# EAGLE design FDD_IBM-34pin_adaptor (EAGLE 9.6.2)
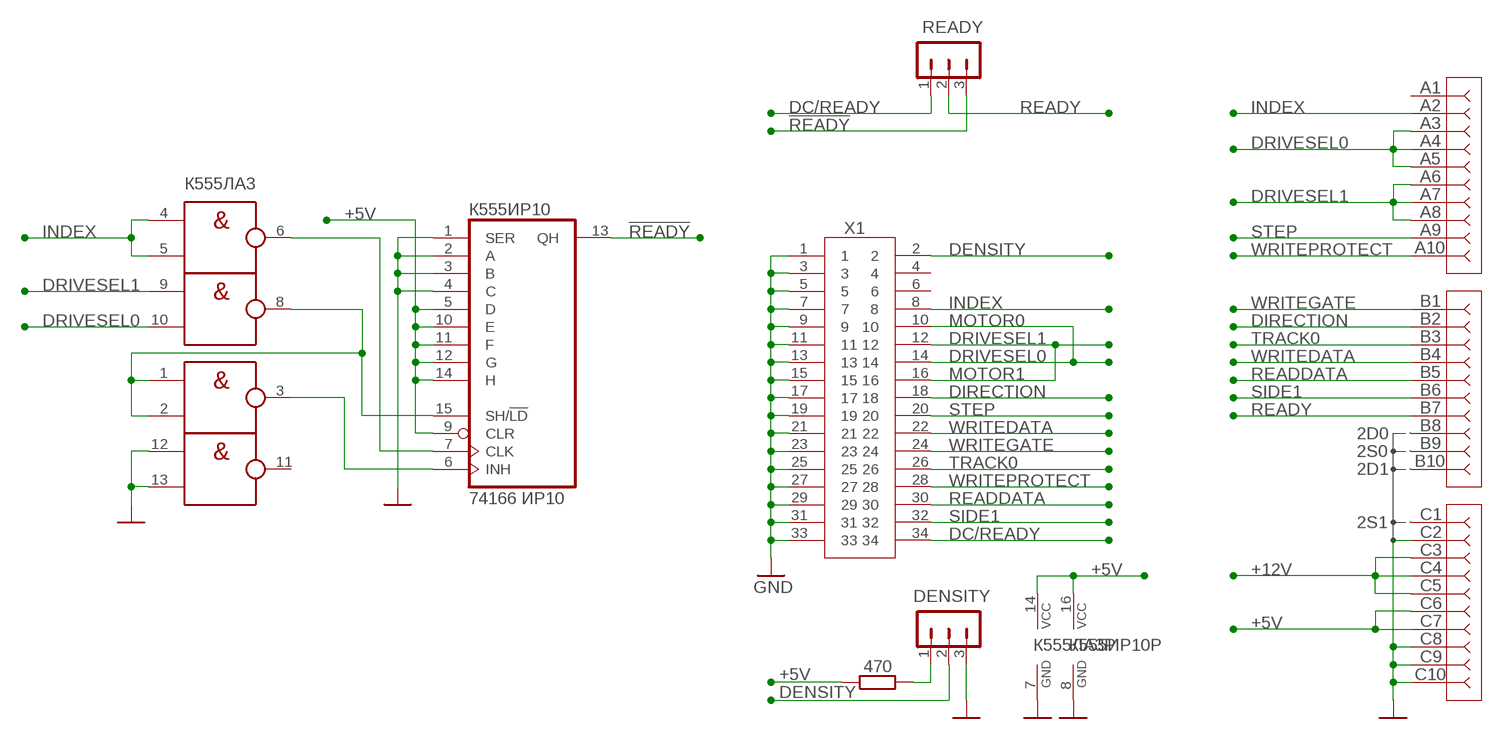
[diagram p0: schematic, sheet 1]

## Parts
DENSITY  JP3S  [JP3S]
R1  470  R-EU_0207/7  [0207/7]
READY  JP3S  [JP3S]
U$2  FDD-30PIN  [FDD-30PIN]
X1  057-034-B  [057-034-1]
К555ИР10  74166 ИР10  74HC166N  [DIL16]
К555ЛА3  К555ЛА3  74LS00N  [DIL14]

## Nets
2D0: U$2.B8
2D1: U$2.B10
2S0: U$2.B9
2S1: U$2.C1
!READY: READY.3 К555ИР10.13(QH)
+5V: R1.1 U$2.C6 U$2.C7 К555ИР10.5(D) К555ИР10.9(CLR) К555ИР10.10(E) К555ИР10.11(F) К555ИР10.12(G) К555ИР10.14(H) К555ИР10.16(VCC) К555ЛА3.14(P:VCC)
+12V: U$2.C3 U$2.C4 U$2.C5
DC/READY: READY.1 X1.34
DENSITY: DENSITY.2 X1.2
DIRECTION: U$2.B2 X1.18
DRIVESEL0: U$2.A3 U$2.A4 U$2.A5 X1.10 X1.14 К555ЛА3.10(C:I1)
DRIVESEL1: U$2.A6 U$2.A7 U$2.A8 X1.12 X1.16 К555ЛА3.9(C:I0)
GND: DENSITY.3 U$2.C2 U$2.C8 U$2.C9 U$2.C10 X1.1 X1.3 X1.5 X1.7 X1.9 X1.11 X1.13 X1.15 X1.17 X1.19 X1.21 X1.23 X1.25 X1.27 X1.29 X1.31 X1.33 К555ИР10.1(SER) К555ИР10.2(A) К555ИР10.3(B) К555ИР10.4(C) К555ИР10.8(GND) К555ЛА3.7(P:GND) К555ЛА3.12(D:I0) К555ЛА3.13(D:I1)
INDEX: U$2.A2 X1.8 К555ЛА3.4(B:I0) К555ЛА3.5(B:I1)
N$1: DENSITY.1 R1.2
N$3: К555ИР10.15(SH/!LD) К555ЛА3.1(A:I0) К555ЛА3.2(A:I1) К555ЛА3.8(C:O)
N$4: К555ИР10.6(INH) К555ЛА3.3(A:O)
N$5: К555ИР10.7(CLK) К555ЛА3.6(B:O)
READDATA: U$2.B5 X1.30
READY: READY.2 U$2.B7
SIDE1: U$2.B6 X1.32
STEP: U$2.A9 X1.20
TRACK0: U$2.B3 X1.26
WRITEDATA: U$2.B4 X1.22
WRITEGATE: U$2.B1 X1.24
WRITEPROTECT: U$2.A10 X1.28
Unconnected: U$2.A1 X1.4 X1.6 К555ЛА3.11(D:O)

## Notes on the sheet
- MOTOR0
- MOTOR1

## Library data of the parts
DENSITY READY = jumpers_lib:JP3S
R1 = rcl:R-EU_: RESISTOR, European symbol; SPICEPREFIX: R
U$2 = AGAT_Slot_Connector:FDD-30PIN
X1 = con-panduit:057-034-: CONNECTOR 34-pin series 057 contact pc board low profile headers
К555ИР10 = 74xx-eu:74*166: 8-bit parallel load SHIFT REGISTER
К555ЛА3 = 74xx-eu:74*00: Quad 2-input NAND gate

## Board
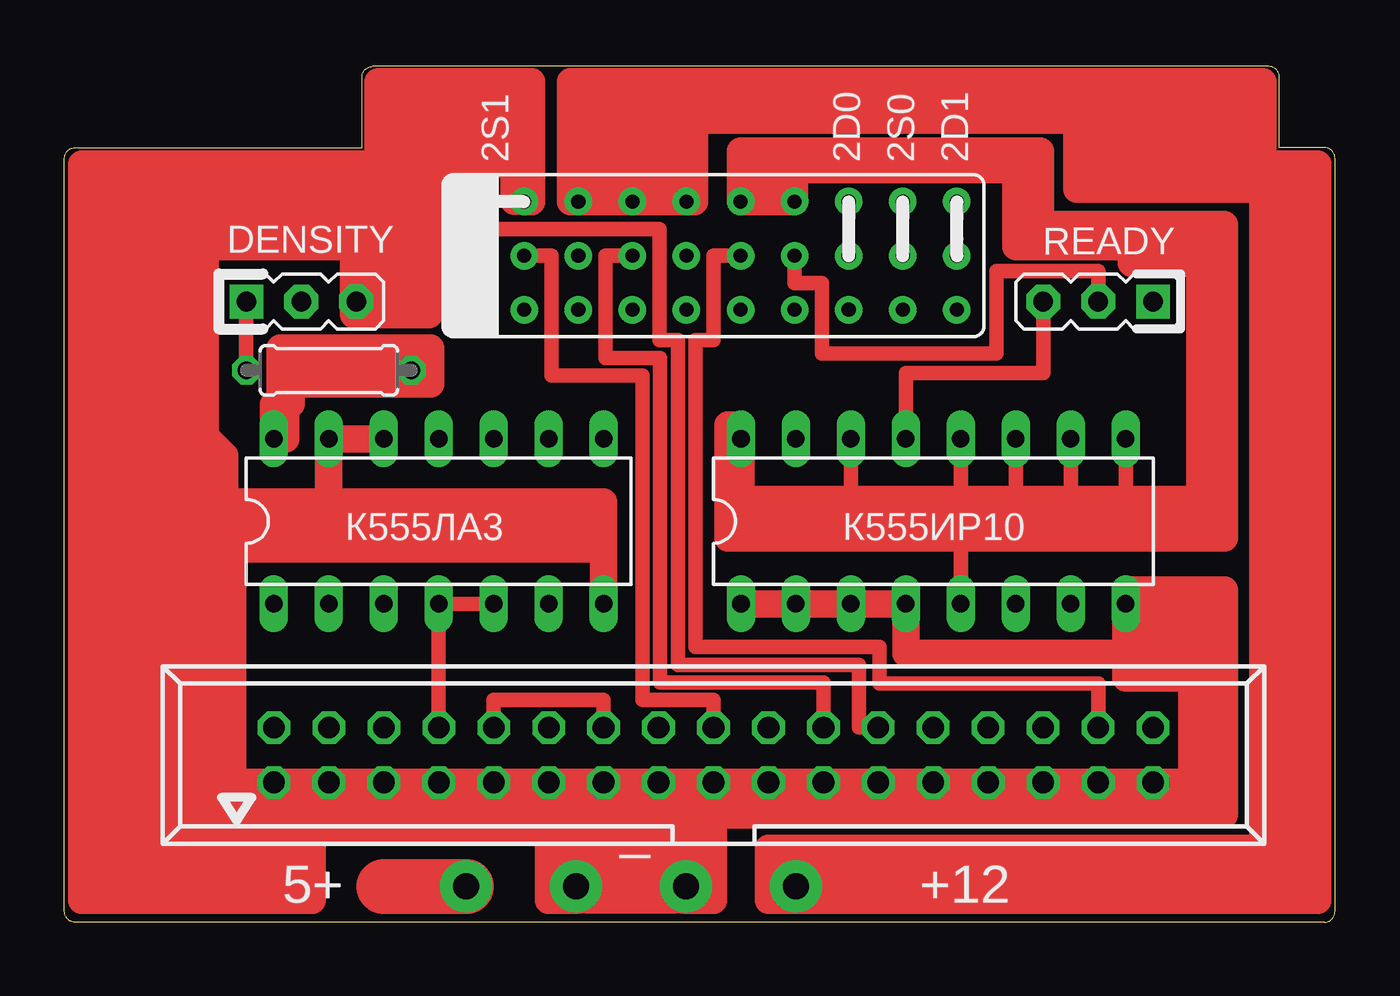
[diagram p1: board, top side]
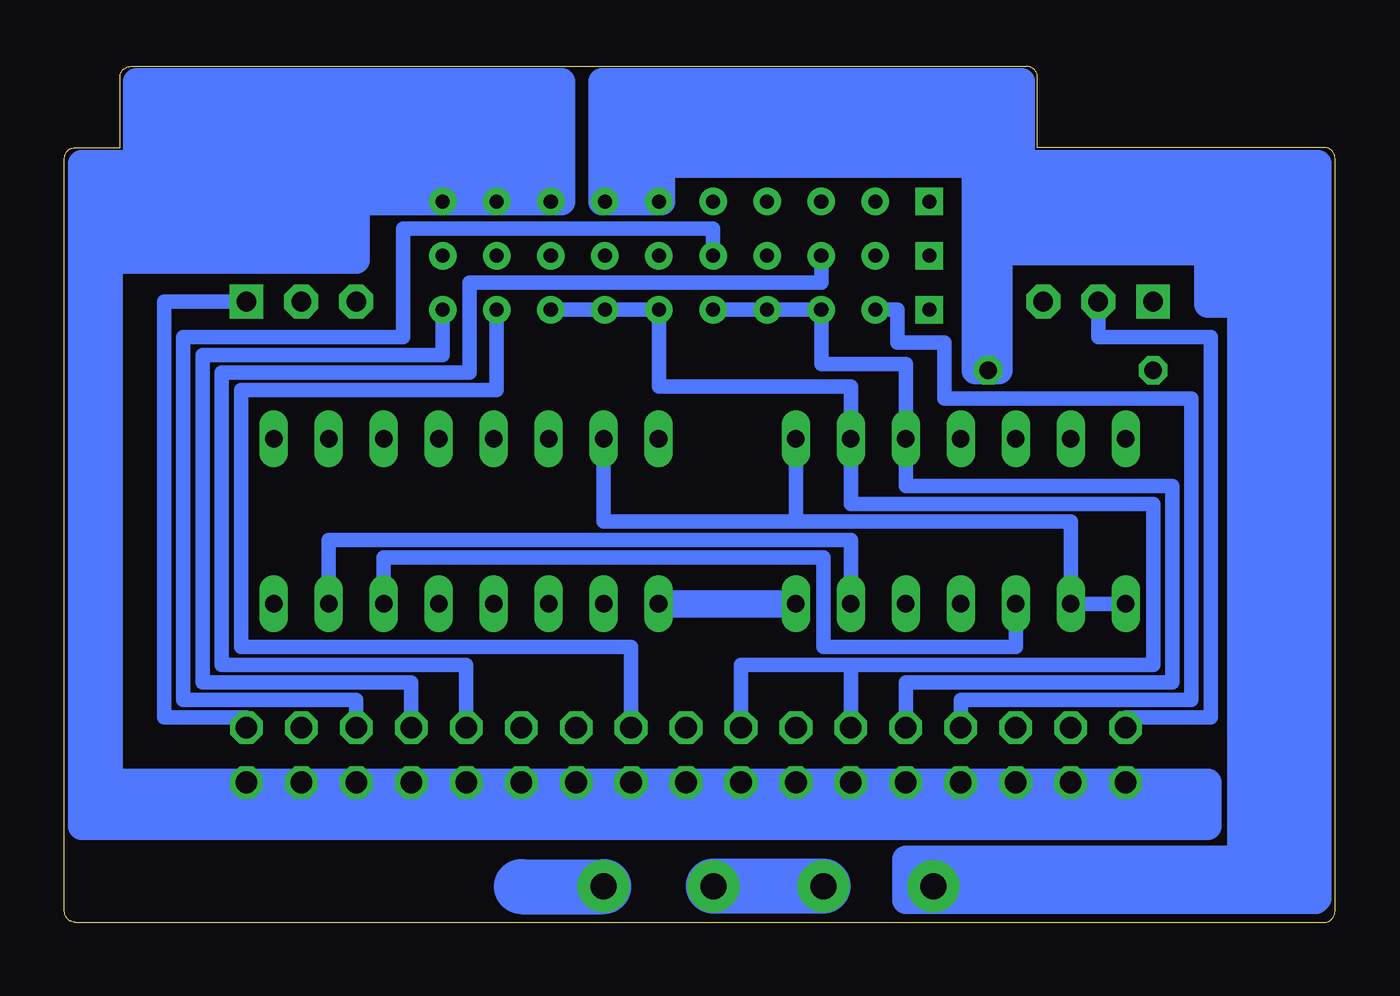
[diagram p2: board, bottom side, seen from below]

Size 58.73 x 39.56 mm. Coordinates in mm from the lower left corner, seen from the top.
Outline: 58.23,0 0.5,0 arc-90 0,0.5 0,35.31 arc-90 0.5,35.81 13.75,35.81 13.75,39.06 arc-90 14.25,39.56 55.66,39.56 arc-90 56.16,39.06 56.16,35.81 58.23,35.81 arc-90 58.73,35.31 58.73,0.5 arc-90 58.23,0
Copper layers (1*16): Top 0.035mm / dielectric 1.5mm / Bottom 0.035mm
Design rules "default *": minimum track width 6mil, minimum drill 0.35mm, track to track 6mil, track to pad 6mil, pad to pad 6mil, via to via 6mil, smd to smd 6mil, copper to edge 0mil, drill to drill 6mil, minimum pad ring 10mil, minimum via ring 8mil, stop-mask expansion 0mil, vias tented up to drill 0mil, thermal gap 10mil

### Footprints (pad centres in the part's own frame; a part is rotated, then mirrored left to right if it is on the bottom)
JP3S = drill 0.914 pad 1.57 square: 1 -2.54,0 | drill 0.914 pad 1.57 octagon: 2 0,0; 3 2.54,0
0207/7 = drill 0.813 octagon: 1 -3.81,0; 2 3.81,0
FDD-30PIN = drill 0.65 pad 1.27 square: A1 -11.25,-2.5; B1 -11.25,0; C1 -11.25,2.5 | drill 0.65 pad 1.27: A2 -8.75,-2.5; A3 -6.25,-2.5; A4 -3.75,-2.5; A5 -1.25,-2.5; A6 1.25,-2.5; A7 3.75,-2.5; A8 6.25,-2.5; A9 8.75,-2.5; A10 11.25,-2.5; B2 -8.75,0; B3 -6.25,0; B4 -3.75,0; B5 -1.25,0; B6 1.25,0; B7 3.75,0; B8 6.25,0; B9 8.75,0; B10 11.25,0; C2 -8.75,2.5; C3 -6.25,2.5; C4 -3.75,2.5; C5 -1.25,2.5; C6 1.25,2.5; C7 3.75,2.5; C8 6.25,2.5; C9 8.75,2.5; C10 11.25,2.5
057-034-1 = drill 1 octagon: 1 -20.32,-1.27; 2 -20.32,1.27; 3 -17.78,-1.27; 4 -17.78,1.27; 5 -15.24,-1.27; 6 -15.24,1.27; 7 -12.7,-1.27; 8 -12.7,1.27; 9 -10.16,-1.27; 10 -10.16,1.27; 11 -7.62,-1.27; 12 -7.62,1.27; 13 -5.08,-1.27; 14 -5.08,1.27; 15 -2.54,-1.27; 16 -2.54,1.27; 17 0,-1.27; 18 0,1.27; 19 2.54,-1.27; 20 2.54,1.27; 21 5.08,-1.27; 22 5.08,1.27; 23 7.62,-1.27; 24 7.62,1.27; 25 10.16,-1.27; 26 10.16,1.27; 27 12.7,-1.27; 28 12.7,1.27; 29 15.24,-1.27; 30 15.24,1.27; 31 17.78,-1.27; 32 17.78,1.27; 33 20.32,-1.27; 34 20.32,1.27
DIL16 = drill 0.813 long: 1 -8.89,-3.81; 2 -6.35,-3.81; 3 -3.81,-3.81; 4 -1.27,-3.81; 5 1.27,-3.81; 6 3.81,-3.81; 7 6.35,-3.81; 8 8.89,-3.81; 9 8.89,3.81; 10 6.35,3.81; 11 3.81,3.81; 12 1.27,3.81; 13 -1.27,3.81; 14 -3.81,3.81; 15 -6.35,3.81; 16 -8.89,3.81
DIL14 = drill 0.813 long: 1 -7.62,-3.81; 2 -5.08,-3.81; 3 -2.54,-3.81; 4 0,-3.81; 5 2.54,-3.81; 6 5.08,-3.81; 7 7.62,-3.81; 8 7.62,3.81; 9 5.08,3.81; 10 2.54,3.81; 11 0,3.81; 12 -2.54,3.81; 13 -5.08,3.81; 14 -7.62,3.81

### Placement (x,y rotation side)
DENSITY  10.95,28.7 0 top
R1  12.22,25.52 180 top
READY  47.78,28.7 180 top
U$2  30,30.82 0 top
X1  30,7.73 0 top
К555ИР10  40.16,18.54 0 top
К555ЛА3  17.3,18.54 0 top

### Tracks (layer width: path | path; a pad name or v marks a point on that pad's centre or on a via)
2D0
  Top 0.61: 36.26,31.6 U$2.B8
2D1
  Top 0.61: 41.26,31.6 U$2.B10
2S0
  Top 0.61: 38.76,31.6 U$2.B9
2S1
  Top 0.61: 19.54,33.31 U$2.C1
!READY
  Top 0.66: К555ИР10.13 38.89,25.39 45.24,25.39 READY.3
+5V  (via drill 1.2 pad 2.4)
  Top 0.66: К555ИР10.14 36.35,19.55 | К555ИР10.12 41.43,19.55 | К555ИР10.11 43.97,19.55 | К555ИР10.10 46.51,19.55 | К555ИР10.9 49.05,19.55 | К555ИР10.5 41.43,17.77
  Top 1.27: 52.48,30.47 52.48,31.24 49.3,31.24 | 52.48,30.47 52.48,19.55 49.05,19.55 46.51,19.55 43.97,19.55 41.43,19.55 36.35,19.55 31.27,19.55 | 31.27,19.55 31.27,18.66 | 53.62,18.66 31.27,18.66 | 31.25,35.66 U$2.C6 32.16,33.31 | 31.25,35.66 33.05,35.66 | 33.05,35.66 45.11,35.66 45.11,32.25 53.62,32.25 53.62,18.66 | 32.16,33.31 33.05,33.31 | 33.05,33.31 U$2.C7 33.75,34.79 43.97,34.79 43.97,31.24 49.3,31.24 | 33.05,35.66 33.05,33.31 | 31.25,35.66 32.16,34.75 32.16,33.31 | 31.27,18.66 31.27,17.77 | 53.62,18.66 53.62,17.77 41.43,17.77 31.27,17.77 | 49.3,31.24 49.3,30.47 52.48,30.47 | 10.21,23.97 10.47,23.97 10.47,24.89 | 10.21,23.97 9.96,23.97 | 10.47,24.89 10.47,25.52 R1.1 | R1.1 16.03,24.89 | 16.03,24.89 10.47,24.89 | R1.1 16.92,25.52 | 16.92,25.52 16.92,24.89 16.03,24.89 | 16.92,25.52 16.92,26.54 9.96,26.54 9.96,23.97 | 9.96,23.97 9.68,23.97 К555ЛА3.14 10.21,22.35 10.21,23.97 | 31.27,19.55 К555ИР10.16 31.27,22.98 30.66,22.98 30.66,17.77 31.27,17.77
  Bottom 1.27: 31.93,33.31 U$2.C6 31.12,33.31 31.12,35.05 16.62,35.05 16.62,31 | 31.93,33.31 32.83,33.31 | 32.83,33.31 U$2.C7 33.88,33.31 33.88,38.87 14.5,38.87 14.5,37.86 | 3.99,32 3.99,34.24 | 2.72,34.24 2.72,35.06 | 3.99,34.24 2.72,34.24 | 2.72,34.24 1.83,34.24 1.83,32.97 1.96,32.97 | 10.09,32.97 3.2,32.97 | 10.09,32.97 10.09,33.14 | 10.09,33.14 10.09,34.12 | 10.09,34.12 10.09,34.24 | 10.09,34.24 10.09,35.06 | 3.99,34.24 6.53,34.24 | 6.53,34.24 10.09,34.24 | 2.72,35.06 6.53,35.06 | 6.53,35.06 10.09,35.06 | 31.93,35.93 31.93,33.31 | 32.83,33.31 32.83,37.86 14.5,37.86 | 6.53,35.06 6.53,34.24 | 10.09,32.97 10.09,32 | 14.5,36.94 14.5,35.93 | 14.5,36.94 14.5,37.86 | 14.5,36.94 31.93,36.94 31.93,35.93 | 31.93,35.93 15.64,35.93 | 15.64,35.93 14.5,35.93 | 16.62,31 15.64,31 15.64,35.93 | 10.09,32 4.6,32 | 4.6,32 3.99,32 | 3.99,32 3.48,32 3.48,31 3.96,31 | 14.62,34.12 14.62,35.06 14.5,35.06 | 14.62,34.12 14.62,33.14 | 14.62,33.14 14.62,32 | 14.62,32 14.62,31 | 10.09,34.12 14.62,34.12 | 14.62,32 10.09,32 | 14.62,33.14 10.09,33.14 | 10.09,35.06 14.5,35.06 | 14.5,35.06 14.5,35.93 | 5.87,31 14.62,31 | 5.87,31 3.96,31 | 19.84,1.66 v18.57,1.66 | 2.72,35.06 0.79,35.06 0.79,1.11 0.88,1.02 19.84,1.02 19.84,1.66 | 1.96,32.97 1.96,1.9 19.84,1.9 | 19.84,1.9 19.84,1.66 | 19.84,1.9 19.84,2.64 | 1.96,32.97 3.2,32.97 | 19.84,2.64 19.84,2.91 3.08,2.91 3.08,28.7 3.2,28.7 | 19.84,2.64 4.35,2.64 4.35,28.57 4.6,28.57 | 3.96,26.54 3.96,27.43 3.2,27.43 3.2,28.7 | 3.2,28.7 3.2,32.97 | 5.87,31 5.87,28.57 4.6,28.57 | 3.96,31 3.96,28.7 | 3.96,28.7 3.96,27.55 | 3.96,28.7 3.2,28.7 | 16.62,31 16.62,27.43 | 14.62,31 15.54,31 15.54,27.43 | 15.54,27.43 16.62,27.43 | 16.62,27.43 16.62,25.52 R1.1 15.54,25.52 15.54,27.43
  Bottom 1.27: 4.6,32 4.6,28.57
+12V  (via drill 1.2 pad 2.4)
  Top 1.27: 27.87,33.31 U$2.C5 29.11,33.31 29.11,37.84 | 27.87,33.31 26.85,33.31 | 26.85,33.31 U$2.C4 | U$2.C4 25.33,33.31 | 25.33,33.31 24.56,33.31 | 24.56,33.31 U$2.C3 | 24.56,33.31 24.56,36.7 | 24.56,36.7 25.33,36.7 | 25.33,33.31 25.33,36.7 | 26.85,33.31 26.85,36.7 | 26.85,36.7 26.25,36.7 | 26.25,36.7 25.33,36.7 | 23.75,36.7 24.56,36.7 | U$2.C3 23.75,36.7 | 26.85,36.7 27.87,36.7 | 27.87,36.7 27.87,37.08 46.79,37.08 | 27.87,36.7 27.87,33.31 | 23.75,37.84 23.75,36.7 | 23.75,37.84 23.75,38.85 | 46.79,37.08 55.4,37.08 | U$2.C4 26.25,36.7 | U$2.C3 23.4,33.32 23.4,38.85 23.75,38.85 | 23.75,37.84 29.11,37.84 | 55.4,37.84 55.4,37.08 | 23.75,38.85 55.4,38.85 55.4,37.84 | 29.11,37.84 55.4,37.84 | 55.4,37.08 55.4,36.06 | 55.4,36.06 55.4,35.05 | 55.4,35.05 56.67,35.05 | 56.67,35.05 57.94,35.05 57.94,3.42 | 57.94,2.91 57.94,1.64 | 57.94,1.64 57.94,1.02 32.54,1.02 32.54,1.64 | 32.54,1.64 32.54,3.42 33.56,3.42 33.56,1.92 v33.81,1.66 | 33.81,2.91 55.4,2.91 | 55.4,2.91 56.67,2.91 | 56.67,2.91 57.94,2.91 | 57.94,3.42 57.94,2.91 | v33.81,1.66 33.79,1.64 32.54,1.64 | v33.81,1.66 34.19,2.05 57.54,2.05 57.94,1.64 | v33.81,1.66 33.81,3.42 57.94,3.42 | 56.67,35.05 56.67,2.91 | 55.4,35.05 55.4,34.92 | 55.4,34.92 55.4,33.9 | 55.4,33.9 55.4,2.91 | 46.79,37.08 46.79,36.06 | 46.79,36.06 46.79,34.92 | 46.79,34.92 46.79,33.9 55.4,33.9 | 46.79,34.92 55.4,34.92 | 46.79,36.06 55.4,36.06
DC/READY
  Bottom 0.66: READY.1 54.13,28.7 54.13,9.47 50.32,9.47 X1.34
DENSITY
  Bottom 0.66: DENSITY.2 10.95,27.04 5.74,27.04 5.74,9.47 9.68,9.47 X1.2
DIRECTION
  Top 0.66: U$2.B2 22.51,30.82 22.51,25.27 26.72,25.27 26.72,10.28 30,10.28 X1.18
DRIVESEL0
  Top 0.66: X1.10 19.84,10.28 24.92,10.28 X1.14
  Bottom 0.66: U$2.A5 U$2.A4 U$2.A3 23.75,25.8 19.84,25.8 К555ЛА3.10 19.84,20.16 7.52,20.16 7.52,11.09 19.84,11.09 X1.10
DRIVESEL1
  Bottom 0.66: U$2.A8 U$2.A7 U$2.A6 31.25,24.76 22.38,24.76 К555ЛА3.9 22.38,19.35 8.41,19.35 8.41,11.91 22.38,11.91 | X1.16 27.46,11.91 22.38,11.91 | X1.12 22.38,11.91
GND  (via drill 1.2 pad 2.4)
  Top 0.61: 41.26,32.52 U$2.C10 | 38.76,32.52 U$2.C9 | 36.26,32.52 U$2.C8 | 21.23,33.33 U$2.C2 20.46,33.31 20.45,33.31
  Top 1.27: 16.03,33.31 16.03,29.96 | 16.03,29.96 16.03,28.95 | 16.03,28.95 16.03,28.09 | 21.25,38.85 U$2.C2 21.59,33.31 21.59,38.85 21.25,38.85 | 21.25,38.85 20.11,38.85 | 20.11,38.85 19.22,38.85 | 18.57,38.85 17.19,38.85 | 17.19,38.85 16.03,38.85 | 16.03,38.85 15.14,38.85 | 14.51,35.05 14.51,38.85 15.14,38.85 | 15.14,38.85 15.14,33.31 | 16.03,33.31 15.14,33.31 | 16.03,33.31 16.03,35.06 | 16.03,35.06 16.03,38.85 | 19.22,35.06 19.22,38.85 | 20.11,35.06 20.11,38.85 | 19.22,38.85 18.19,38.85 18.19,35.85 | DENSITY.3 13.49,28.95 | 13.49,28.95 13.49,29.96 | 13.49,29.96 14.25,29.96 | 15.14,29.96 16.03,29.96 | 20.11,35.06 20.79,35.06 20.79,33.33 21.23,33.33 | 16.84,35.06 17.19,35.06 | 17.19,35.06 19.22,35.06 | 19.22,35.06 20.11,35.06 | 17.19,38.85 17.19,35.06 | 16.84,35.06 16.03,35.06 | X1.17 X1.19 X1.21 X1.23 X1.25 X1.27 X1.29 X1.31 X1.33 52.11,6.46 | X1.17 X1.15 X1.13 X1.11 | X1.11 X1.9 X1.7 X1.5 X1.3 X1.1 7.77,6.46 | К555ЛА3.7 24.92,17.27 | 7.77,17.27 24.92,17.27 | 7.77,17.27 7.77,6.46 | 52.11,6.46 52.86,6.46 | 52.86,15.36 52.86,6.46 | DENSITY.3 13.49,28.09 | 13.49,28.09 13.36,28.09 13.36,32.76 12.86,32.76 | 6.5,31.24 5.36,31.24 | 5.87,6.46 5.36,6.46 5.36,31.24 | 5.87,6.46 6.63,6.46 6.63,17.27 | 7.14,6.46 7.77,6.46 | 7.77,17.27 6.63,17.27 | 6.63,17.27 6.38,17.27 6.38,22.6 6.5,22.47 | 6.5,22.47 6.5,31.24 | 13.49,35.05 14.51,35.05 | 13.49,29.96 13.49,31.24 | 13.49,31.24 13.49,32.12 | 13.49,32.12 13.49,33.77 | 13.49,33.77 13.49,35.05 | 15.14,33.31 15.14,29.96 | 14.51,35.05 14.51,32.38 14.25,32.38 14.25,29.96 | 14.25,29.96 15.14,29.96 | 13.49,35.05 12.86,35.05 | 12.86,32.76 12.86,35.05 | 16.84,28.7 DENSITY.3 | 16.84,28.7 16.84,35.06 | 24.92,17.27 24.92,18.28 | 24.92,18.28 7.39,18.28 7.39,19.42
  Top 1.27: 6.5,22.47 7.39,21.58 7.39,19.42 | 52.11,6.46 52.11,11.3 | 52.11,11.3 52.11,12.44 | 51.59,14.09 52.11,14.09 52.11,12.44 | 51.59,14.09 49.05,14.09 | 52.86,15.36 53.62,15.36 53.62,6.46 | 53.62,6.46 53.62,5.45 | 53.62,6.46 52.86,6.46 | 5.87,6.46 5.87,5.84 | 5.87,5.84 5.87,5.45 11.46,5.45 | 5.87,5.84 4.98,5.84 4.98,4.31 22.38,4.31 | 11.46,5.45 53.62,5.45 | 52.86,15.36 49.05,15.36 | 22.38,2.28 22.38,1.02 23.65,1.02 v23.65,1.66 23.65,1.03 28.73,1.03 v28.73,1.66 28.73,1.02 30,1.02 30,2.28 | 22.38,2.28 22.38,3.3 | 22.38,3.3 22.38,4.31 | 22.38,4.31 X1.11 | 30,2.28 30,3.3 | 30,3.3 30,4.31 | 30,4.31 30,4.97 | 30,4.97 X1.17 | 22.38,2.28 30,2.28 | 22.38,4.31 30,4.31 | 22.38,3.3 30,3.3 | 53.62,5.45 53.62,4.97 30,4.97 | 11.46,2.15 11.46,1.02 0.79,1.02 0.79,35.05 12.86,35.05 | 11.46,2.15 11.46,3.3 | 11.46,3.3 11.46,5.45 | 13.49,33.77 1.55,33.77 1.55,2.15 11.46,2.15 | 12.86,32.76 2.7,32.76 2.7,2.91 3.58,2.91 3.58,32.12 13.49,32.12 | 11.46,3.3 4.22,3.3 4.22,31.24 5.36,31.24 | 13.49,31.24 6.5,31.24 | 16.03,28.09 13.49,28.09 | 13.49,28.95 16.03,28.95 | 24.92,18.28 24.92,19.42 12.22,19.42 | 7.39,19.42 12.22,19.42 | К555ЛА3.12 К555ЛА3.13 12.22,19.42 | 16.03,28.09 16.84,28.09 16.84,28.7 | К555ИР10.8 49.05,13.46 | 49.05,13.46 49.05,12.44 | 49.05,12.44 38.89,12.44 К555ИР10.4 К555ИР10.3 К555ИР10.2 К555ИР10.1 | 49.05,12.44 52.11,12.44 | 51.59,14.09 51.59,13.46 49.05,13.46 | 49.05,12.44 49.05,11.3 52.11,11.3
  Bottom 1.27: U$2.C10 U$2.C9 U$2.C8 35.74,33.31 35.74,34.56 | 35.74,35.06 35.74,35.94 | 35.74,34.56 35.74,35.06 | 41.38,34.06 41.38,33.31 U$2.C10 | 41.25,34.56 41.25,35.06 | 35.74,34.56 41.25,34.56 | 41.25,34.56 41.38,34.56 41.38,34.06 | 35.74,35.06 41.25,35.06 | 35.74,37.81 35.74,38.86 55.4,38.86 55.4,37.81 | 35.74,37.81 35.74,36.94 | 35.74,36.94 35.74,35.94 | 41.25,35.06 55.4,35.06 | 54.73,33.77 54.73,33.31 U$2.C10 | 54.73,33.77 54.73,34.06 | 54.73,34.06 54.73,34.16 56.92,34.16 56.92,29.96 56.67,29.96 | 54.73,34.06 45.24,34.06 | 45.24,34.06 41.38,34.06 | 55.4,36.94 55.4,35.94 | 55.4,35.94 55.4,35.06 | 35.74,37.81 55.4,37.81 | 55.4,36.94 55.4,37.81 | 35.74,36.94 55.4,36.94 | 35.74,35.94 55.4,35.94 | X1.1 X1.3 X1.5 X1.7 X1.9 X1.11 X1.13 X1.15 X1.17 X1.19 X1.21 X1.23 X1.25 X1.27 X1.29 X1.31 X1.33 56.67,6.46 | 45.24,34.06 45.24,32.51 | 45.24,32.51 45.24,31.36 | 45.24,31.36 45.24,30.6 55.78,30.6 | 55.78,30.6 56.67,30.6 56.67,29.96 | 56.67,29.96 56.67,6.46 | 56.67,6.46 57.94,6.46 | 57.94,6.46 57.94,35.06 55.4,35.06 | 54.73,33.77 55.78,33.77 55.78,32.51 | 55.78,32.51 55.78,30.6 | 45.24,32.51 55.78,32.51 | 45.24,31.36 56.54,31.36 | 57.94,6.46 57.94,5.33 | 57.94,5.33 8.79,5.33 8.79,5.58 X1.1 | 57.94,5.33 57.94,4.44 8.41,4.44 | 8.41,4.44 8.41,5.33 | 8.41,5.33 8.41,6.46 | X1.1 8.41,6.46 | 8.41,6.46 5.87,6.46 5.87,5.33 | 8.41,4.44 5.87,4.44 5.87,5.33 | 5.87,5.33 8.41,5.33 | К555ИР10.1 К555ЛА3.7
  Bottom 2.54: v23.65,1.66 v28.73,1.66
INDEX
  Top 0.66: X1.8 К555ЛА3.4 К555ЛА3.5
  Bottom 0.66: X1.8 17.3,10.28 6.63,10.28 6.63,24.2 18.06,24.2 18.06,26.79 20.23,26.79 20.23,28.32 U$2.A2
N$1
  Top 0.66: R1.2 DENSITY.1
N$2
  Top 2.54: 18.57,1.64 14.76,1.64
N$3
  Bottom 0.66: К555ЛА3.1 К555ЛА3.2 12.22,18.54 24.92,18.54 | К555ЛА3.8 24.92,18.54 | К555ИР10.15 33.81,18.54 24.92,18.54
N$4
  Bottom 0.66: К555ЛА3.3 14.76,12.72 23.65,12.72 23.65,16.86 43.97,16.86 К555ИР10.6
N$5
  Bottom 0.66: К555ЛА3.6 22.38,17.67 46.51,17.67 К555ИР10.7
N$9
  Bottom 2.54: 37.62,1.64 33.81,1.64
READDATA
  Bottom 0.66: U$2.B5 28.75,32.06 43.08,32.06 43.08,27.04 53.24,27.04 53.24,10.28 45.24,10.28 X1.30
READY
  Top 0.66: U$2.B7 33.75,29.56 35,29.56 35,26.28 43.08,26.28 43.08,30.09 47.78,30.09 READY.2
SIDE1
  Top 0.66: X1.32 47.78,11.04 37.67,11.04 37.67,12.72 29.16,12.72 29.16,26.92 30,26.92 30,30.82 U$2.B6
STEP
  Bottom 0.66: U$2.A9 38.75,24.61 50.57,24.61 50.57,12.72 32.54,12.72 X1.20
TRACK0
  Bottom 0.66: U$2.B3 23.75,29.56 40,29.56 40,25.42 51.46,25.42 51.46,11.91 40.16,11.91 X1.26
WRITEDATA
  Top 0.66: X1.22 35.08,11.09 27.54,11.09 27.54,26.08 25.01,26.08 25.01,30.82 U$2.B4
WRITEGATE
  Top 0.66: U$2.B1 18.75,32.05 27.46,32.05 27.46,32.03 27.49,32.03 27.49,26.92 28.35,26.92 28.35,11.91 36.73,11.91 36.73,9 X1.24
WRITEPROTECT
  Bottom 0.66: U$2.A10 41.25,26.23 52.35,26.23 52.35,11.09 42.7,11.09 X1.28

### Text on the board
tPlace: 2S1 | 2D0 | 2S0 | 2D1 | _ | 5+ | +12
